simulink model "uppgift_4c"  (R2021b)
settings: Solver=VariableStepAuto  StartTime=0.0  StopTime=10.0  RelTol=1e-3
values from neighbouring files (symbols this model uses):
  AFs = 14.6    [Lektion_2.m]
  eta_vol = 0.8    [Lektion_2.m]
  m_dot_a_end = 18*1e-3    (= 0.018)    [Lektion_2.m]
  m_dot_a_start = 12*1e-3    (= 0.012)    [Lektion_2.m]
  m_dot_fi_start = m_dot_a_start/AFs    (= 0.000821917808219)    [Lektion_2.m]
  n_cyl = 4    [Lektion_2.m]
  N_init = 3000/60    (= 50)    [Lektion_2.m]
  n_r = 2    [Lektion_2.m]
  p_im_init = 40*1e3    (= 40000)    [Lektion_2.m]
  R = 280    [Lektion_2.m]
  T_i = 320    [Lektion_2.m]
  tau_th = 1/0.1    (= 10)    [Lektion_2.m]
  V_d = 0.55/1e3    (= 0.00055)    [Lektion_2.m]
  V_i = 2/1e3    (= 0.002)    [Lektion_2.m]

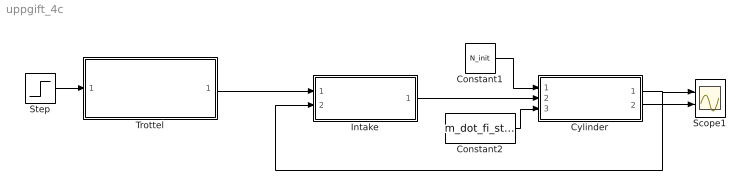
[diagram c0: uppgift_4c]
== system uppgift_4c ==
  Constant1 : Constant  Value=N_init
  Constant2 : Constant  Value=m_dot_fi_start
  Cylinder : Subsystem
  Intake : Subsystem
  Scope1 : Scope  NumInputPorts=2
  Step : Step  Time=3  Before=m_dot_a_start  After=m_dot_a_end  SampleTime=0
  Trottel : Subsystem
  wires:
  Cylinder/1(m_ac [kg/s]) -> Intake/2(m_ac [kg/s]), Scope1/1
  Step/1 -> Trottel/1(m_at,raf [kg/s])
  Trottel/1(m_at [kg/s]) -> Intake/1(m_at [kg/s])
  Cylinder/2(lambda_c [-]) -> Scope1/2
  Intake/1(p_im [Pa]) -> Cylinder/2(p_im [Pa])
  Constant1/1 -> Cylinder/1(N [rps])
  Constant2/1 -> Cylinder/3(m_fi [kg/s])

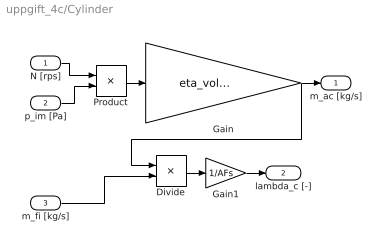
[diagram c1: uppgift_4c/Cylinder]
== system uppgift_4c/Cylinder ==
  N [rps] : Inport
  p_im [Pa] : Inport  Port=2
  m_fi [kg/s] : Inport  Port=3
  Divide : Product  Inputs=*/
  Gain : Gain  Gain=eta_vol*V_d*n_cyl/(n_r*R*T_i)
  Gain1 : Gain  Gain=1/AFs
  Product : Product
  m_ac [kg/s] : Outport
  lambda_c [-] : Outport  Port=2
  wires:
  N [rps]/1 -> Product/1
  p_im [Pa]/1 -> Product/2
  Product/1 -> Gain/1
  Gain/1 -> Divide/1, m_ac [kg/s]/1
  m_fi [kg/s]/1 -> Divide/2
  Divide/1 -> Gain1/1
  Gain1/1 -> lambda_c [-]/1

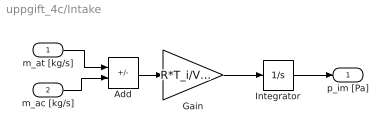
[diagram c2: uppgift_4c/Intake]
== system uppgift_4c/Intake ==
  m_at [kg/s] : Inport
  m_ac [kg/s] : Inport  Port=2
  Add : Sum  Inputs=+-
  Gain : Gain  Gain=R*T_i/V_i
  Integrator : Integrator  InitialCondition=p_im_init
  p_im [Pa] : Outport
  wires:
  Integrator/1 -> p_im [Pa]/1
  Gain/1 -> Integrator/1
  m_ac [kg/s]/1 -> Add/2
  m_at [kg/s]/1 -> Add/1
  Add/1 -> Gain/1

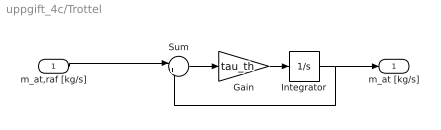
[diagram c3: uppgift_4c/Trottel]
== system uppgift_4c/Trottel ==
  m_at,raf [kg/s] : Inport
  Gain : Gain  Gain=tau_th
  Integrator : Integrator  InitialCondition=m_dot_a_start
  Sum : Sum  Inputs=|+-
  m_at [kg/s] : Outport
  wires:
  Sum/1 -> Gain/1
  Integrator/1 -> m_at [kg/s]/1, Sum/2
  m_at,raf [kg/s]/1 -> Sum/1
  Gain/1 -> Integrator/1
